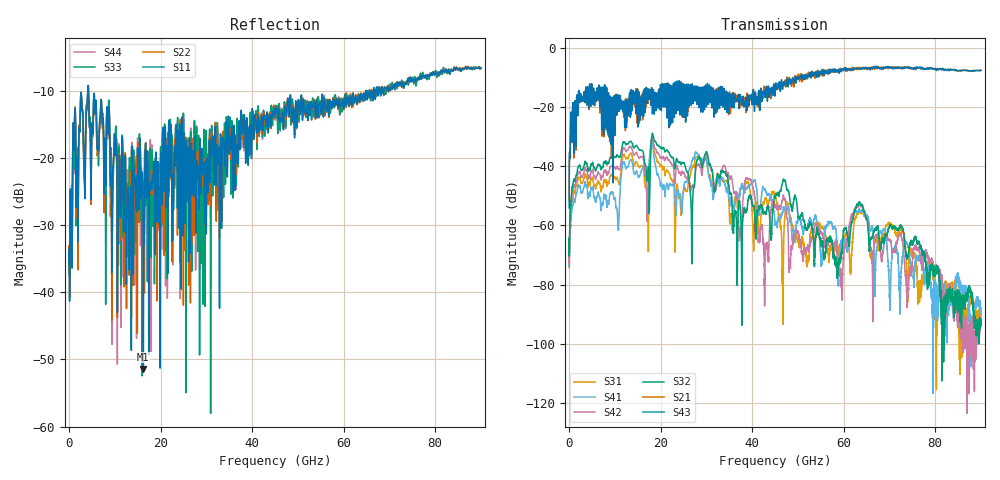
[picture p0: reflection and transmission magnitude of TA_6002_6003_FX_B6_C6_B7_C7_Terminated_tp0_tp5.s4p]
!Touchstone File created by Channel Assembly Engine (Version 2.0.0_Beta1)
!Current time:  2022 6/29 11:28:37
# Hz S RI R 50
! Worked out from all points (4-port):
!   9000 points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, 10 MHz to 90 GHz, reference 50 ohm
!   strongest paths, dB at 10 MHz, 22.51 GHz, 45.01 GHz, 67.51 GHz, 90 GHz:
!     S43: -54.1, -15.7, -15.8, -6.9, -7.5
!     S21: -51.4, -13.5, -13.3, -6.7, -7.6
!     S32: -66.2, -37.1, -50.6, -60.7, -92.2
!     S42: -66.4, -39.5, -53.8, -63.1, -94.0
!     S41: -68.1, -46.5, -59.2, -64.2, -90.0
!     S31: -65.2, -44.8, -50.5, -64.3, -90.3
!   lowest |S11| = -51.4 dB at 16.23 GHz (marker M1), VSWR 1.01, Z = 49.7 - j0.02 ohm
!   |S11| at or under -10 dB: start of sweep to 4.072 GHz; 4.262 GHz to 64.87 GHz (60.61 GHz wide, 175 % of centre); 65.46 GHz to 66.03 GHz (573.3 MHz wide, 0.872 % of centre)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
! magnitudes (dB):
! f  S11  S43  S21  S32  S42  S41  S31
! 10 MHz  -34.0  -54.1  -51.4  -66.2  -66.4  -68.1  -65.2
! 2.45 GHz  -13.2  -15.8  -16.3  -40.2  -42.5  -47.5  -44.5
! 16.23 GHz  -51.4  -21.3  -14.6  -35.4  -37.4  -39.9  -40.1
! 39.44 GHz  -15.2  -16.8  -16.7  -50.0  -44.2  -46.5  -47.3
! 43.1 GHz  -15.0  -13.0  -13.5  -55.8  -66.5  -48.7  -51.3
! 63.72 GHz  -10.4  -7.1  -6.7  -53.0  -53.6  -55.5  -55.8
! 90 GHz  -6.5  -7.5  -7.6  -92.2  -94.0  -90.0  -90.3
